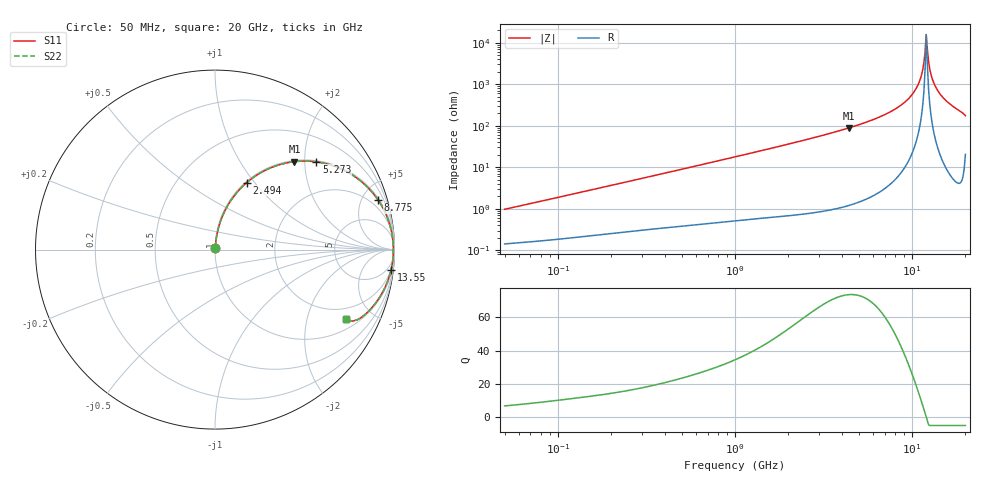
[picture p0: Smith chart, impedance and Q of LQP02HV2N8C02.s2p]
!Murata Part Number: LQP02HV2N8C02
!These Parameters are Measured in Series Mode Connection
!  o--[Z]--o
!Port1  Port2
!  o-------o
!Freq. Start=50[MHz] Stop=20[GHz], 401[Steps]
# Hz S RI R 50
!Freq.(Hz) S11(Real) S11(Imag) S21(Real) S21(Imag) S12(Real) S12(Imag) S22(Real) S22(Imag)
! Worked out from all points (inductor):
!   401 points, 50 MHz to 20 GHz, reference 50 ohm
!   read as one part in series: L = 3.03 nH near 51.52 MHz
!   highest Q = 73.7 at 4.406 GHz (marker M1), where L = 3.21 nH
!   self-resonance near 12.02 GHz
!   S11 on the Smith chart (normalised r, x): 50 MHz: 1.00, +0.02; 2.494 GHz: 1.02, +0.91; 5.273 GHz: 1.03, +2.28; 8.775 GHz: 1.16, +6.53; 13.55 GHz: 2, -18; 20 GHz: 1.41, -3.47
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5e7  0.00152 0.0096  0.9985 -0.0096  0.9985 -0.0096  0.00152 0.0096
1.364002e8  0.00276 0.0251  0.9972 -0.0251  0.9972 -0.0251  0.00276 0.0251
3.721004e8  0.00777 0.0662  0.9922 -0.0662  0.9922 -0.0662  0.00777 0.0662
1e9  0.0353 0.1706  0.9647 -0.1706  0.9647 -0.1706  0.0353 0.1706
2.493527e9  0.1764 0.3729  0.8236 -0.3729  0.8236 -0.3729  0.1764 0.3729
2.728004e9  0.2059 0.3966  0.7941 -0.3966  0.7941 -0.3966  0.2059 0.3966
4.405649e9  0.4423 0.4899  0.5577 -0.4899  0.5577 -0.4899  0.4423 0.4899
5.273168e9  0.5643 0.489  0.4357 -0.489  0.4357 -0.489  0.5643 0.489
7.442007e9  0.8113 0.3824  0.1887 -0.3824  0.1887 -0.3824  0.8113 0.3824
8.774992e9  0.9088 0.2759  0.0912 -0.2759  0.0912 -0.2759  0.9088 0.2759
9.892087e9  0.9597 0.1792  0.0403 -0.1792  0.0403 -0.1792  0.9597 0.1792
1.082228e10  0.9835 0.0991  0.0165 -0.0991  0.0165 -0.0991  0.9835 0.0991
1.131968e10  0.9903 0.0575  0.00969 -0.0575  0.00969 -0.0575  0.9903 0.0575
1.166392e10  0.9929 0.0294  0.00714 -0.0294  0.00714 -0.0294  0.9929 0.0294
1.183995e10  0.9935 0.0153  0.00647 -0.0153  0.00647 -0.0153  0.9935 0.0153
1.201863e10  0.9938 0.0012  0.00619 -0.0012  0.00619 -0.0012  0.9938 0.0012
1.238412e10  0.9931 -0.027  0.00685 0.027  0.00685 0.027  0.9931 -0.027
1.257102e10  0.9922 -0.0411  0.00779 0.0411  0.00779 0.0411  0.9922 -0.0411
1.295331e10  0.9891 -0.0692  0.0109 0.0692  0.0109 0.0692  0.9891 -0.0692
1.354865e10  0.9815 -0.1109  0.0185 0.1109  0.0185 0.1109  0.9815 -0.1109
1.573793e10  0.9315 -0.2416  0.0685 0.2416  0.0685 0.2416  0.9315 -0.2416
2e10  0.7301 -0.3889  0.2699 0.3889  0.2699 0.3889  0.7301 -0.3889
